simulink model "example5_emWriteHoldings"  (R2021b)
settings: Solver=FixedStepAuto  StartTime=0  StopTime=inf  FixedStep=0.5  RelTol=1e-3  EnableMultiTasking=on
undefined symbols (not defined in the file or in its folder): based, classic, dsPic33, MCC, Microchip, PIC24
libraries: emMBSlaveLib x5, simulink x1, embeddedCreatorLib x1

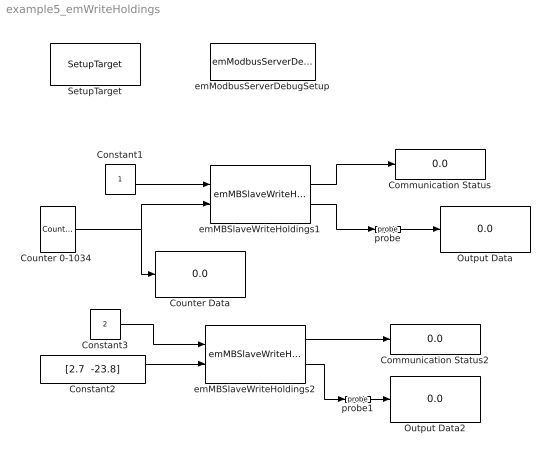
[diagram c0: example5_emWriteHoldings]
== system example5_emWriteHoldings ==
  Communication Status : Display
  Communication Status2 : Display
  Constant1 : Constant  OutDataTypeStr=uint16
  Constant2 : Constant  Value="[2.7  -23.8]"  OutDataTypeStr=single
  Constant3 : Constant  Value=2  OutDataTypeStr=uint16
  "Counter 0-1034 " : simulink/Sources/Counter Limited  uplimit=1034  tsamp=-1
  Counter Data : Display
  Output Data : Display
  Output Data2 : Display
  SetupTarget : embeddedCreatorLib/SetupTarget  Tag=SetupTarget  Priority=0  c_platform=Microchip PIC24/dsPic33 based on MCC classic  c_debug=on
  emMBSlaveWriteHoldings1 : emMBSlaveLib/emMBSlaveWriteHoldings  c_ServerID=1  c_UartNo=1  c_OutputDataType=uint16  c_wordOrder=big-endian  c_factor=1x  c_minAdr=1  c_RegQTY=10  c_singleWriting=off  c_DataPortType=uint16  c_sampleTime=-1
  emMBSlaveWriteHoldings2 : emMBSlaveLib/emMBSlaveWriteHoldings  c_ServerID=1  c_UartNo=1  c_OutputDataType=int32  c_wordOrder=big-endian  c_factor=10x  c_minAdr=1  c_RegQTY=10  c_singleWriting=on  c_DataPortType=single  c_sampleTime=-1
  emModbusServerDebugSetup : emMBSlaveLib/emModbusServerDebugSetup  Tag=emModbusSlaveSetup  c_objID=0  c_uartNo=2  c_baudrate=19200  c_serverID=1  c_baudrate4PC=19200  c_forceLongerSpace=on  c_holdingRegsQTY=10  c_minHoldingAddr=1  c_inputRegsQTY=0  c_minInputRegAddr=1  c_coilRegsQTY=0  c_minCoilAddr=8  c_discreteRegsQTY=0  c_minDiscreteAddr=8  c_enableDebug=on  c_breakpointMaxQTY=100  c_probeMaxWordQTY=200  c_emWaitQTY=0  g_COMPortNo=COM5  c_Name_method=By physical port name and bit number  c_PortName=B  c_BitNo=11  c_TxEnable485="\"LATBbits.LATB11\""  c_TxEnable485Polarity=on
  probe : emMBSlaveLib/probe  Tag=emProbe  c_ObjID=1  c_serverID=1  c_UartNo=1  c_StartAddr=6  c_ConstantDataSource=off
  probe1 : emMBSlaveLib/probe  Tag=emProbe  c_ObjID=0  c_serverID=1  c_UartNo=1  c_StartAddr=2  c_ConstantDataSource=off
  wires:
  Constant1/1 -> emMBSlaveWriteHoldings1/1
  emMBSlaveWriteHoldings1/1 -> Communication Status/1
  "Counter 0-1034 "/1 -> emMBSlaveWriteHoldings1/2, Counter Data/1
  emMBSlaveWriteHoldings1/2 -> probe/1
  probe/1 -> Output Data/1
  Constant2/1 -> emMBSlaveWriteHoldings2/2
  Constant3/1 -> emMBSlaveWriteHoldings2/1
  emMBSlaveWriteHoldings2/1 -> Communication Status2/1
  probe1/1 -> Output Data2/1
  emMBSlaveWriteHoldings2/2 -> probe1/1
